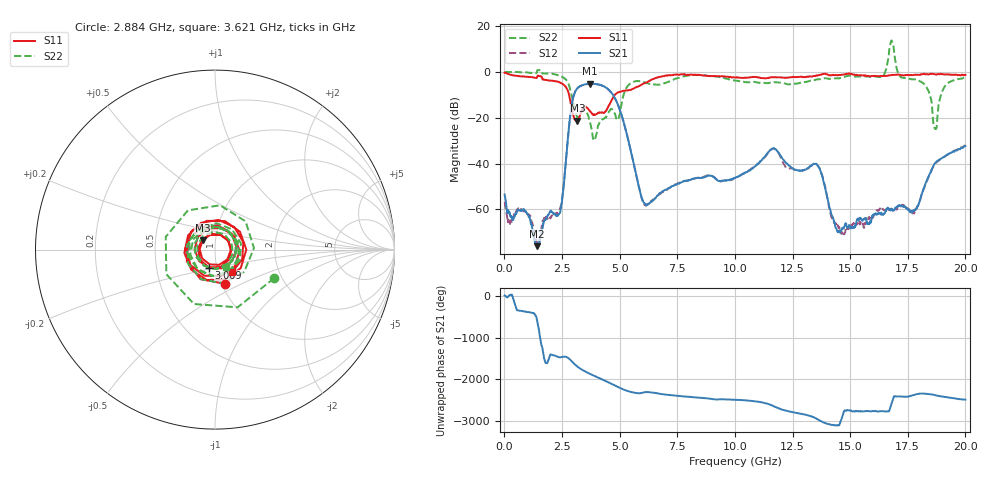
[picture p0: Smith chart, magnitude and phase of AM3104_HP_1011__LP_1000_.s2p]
!Created with skrf (http://scikit-rf.org).
# Hz S RI R 50.0
!freq ReS11 ImS11 ReS21 ImS21 ReS12 ImS12 ReS22 ImS22
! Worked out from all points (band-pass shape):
!   1601 points, 10 MHz to 20 GHz, reference 50 ohm
!   highest |S21| = -5.14 dB at 3.721 GHz (marker M1); lowest = -76.0 dB at 1.422 GHz (marker M2)
!   |S21| within 3 dB of the highest: 3.096 GHz to 4.56 GHz (1.464 GHz wide, 38.2 % of centre)
!   lowest |S11| = -21.3 dB at 3.171 GHz (marker M3), VSWR 1.19, Z = 43.4 + j4.49 ohm
!   |S11| at or under -10 dB: 2.805 GHz to 4.797 GHz (1.992 GHz wide, 52.4 % of centre)
!   |S22| runs from -29.4 to 13.7 dB; largest |S21 - S12| = 0.042
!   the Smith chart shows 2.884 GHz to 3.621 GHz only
!   S11 on the Smith chart (normalised r, x): 2.884 GHz: 1.03, -0.41; 3.009 GHz: 0.92, -0.18; 3.621 GHz: 1.17, -0.30
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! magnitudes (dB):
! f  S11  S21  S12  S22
! 10 MHz  -0.4  -53.5  -56.8  0.0
! 1.422 GHz  -2.3  -76.0  -75.0  0.4
! 2.421 GHz  -4.7  -61.3  -59.2  -1.8
! 2.884 GHz  -14.1  -17.0  -17.1  -8.7
! 3.009 GHz  -19.5  -10.3  -10.4  -14.3
! 3.171 GHz  -21.3  -7.1  -7.2  -19.9
! 3.346 GHz  -17.3  -5.9  -6.0  -17.5
! 3.621 GHz  -16.0  -5.3  -5.4  -18.7
! 3.721 GHz  -17.2  -5.1  -5.2  -22.1
! 4.883 GHz  -9.2  -13.3  -13.4  -20.8
! 6.057 GHz  -5.1  -57.1  -57.8  -4.5
! 6.682 GHz  -2.3  -53.6  -53.6  -5.6
! 10.01 GHz  -2.5  -46.3  -46.3  -3.8
! 11.64 GHz  -2.4  -33.5  -33.5  -4.5
! 13.34 GHz  -2.1  -40.7  -40.7  -3.8
! 14.49 GHz  -1.4  -69.6  -67.8  -2.8
! 16.68 GHz  -1.6  -59.6  -60.2  7.3
! 17.79 GHz  -1.3  -60.6  -61.5  -3.2
! 18.38 GHz  -1.2  -46.2  -46.6  -7.9
! 18.69 GHz  -1.1  -39.7  -39.9  -24.8
! 19.1 GHz  -1.2  -36.8  -36.9  -6.5
! 20 GHz  -1.3  -32.4  -32.1  -2.6
